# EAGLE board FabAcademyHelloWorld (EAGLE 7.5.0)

Size 100 x 80 mm. Coordinates in mm from the lower left corner, seen from the top.
Outline: 0,0 100,0 100,80 0,80 0,0
Copper layers (1*16): Top 0.035mm / dielectric 1.5mm / Bottom 0.035mm
Design rules "default": minimum track width 10mil, minimum drill 24mil, track to track 8mil, track to pad 8mil, pad to pad 8mil, via to via 8mil, smd to smd 8mil, copper to edge 40mil, drill to drill 8mil, minimum pad ring 10mil, minimum via ring 8mil, stop-mask expansion 4mil, vias tented up to drill 0mil, thermal gap 10mil

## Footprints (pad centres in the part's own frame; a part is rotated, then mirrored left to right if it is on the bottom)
C1206FAB = smd 1.27 x 1.905: 1 -1.651,0; 2 1.651,0
SOIC14 = smd 0.61 x 2.21: 1 -3.81,-2.603; 2 -2.54,-2.603; 3 -1.27,-2.603; 4 0,-2.603; 5 1.27,-2.603; 6 2.54,-2.603; 7 3.81,-2.603; 8 3.81,2.603; 9 2.54,2.603; 10 1.27,2.603; 11 0,2.603; 12 -1.27,2.603; 13 -2.54,2.603; 14 -3.81,2.603
1X02 = drill 1.016 pad 1.88: 1 0,0; 2 2.54,0
R1206FAB = smd 1.27 x 1.905: 1 -1.651,0; 2 1.651,0
6MM_SWITCH = smd 2.286 x 1.524: 1 -3.302,2.286; 2 3.302,2.286; 3 -3.302,-2.286; 4 3.302,-2.286
2X03SMD = smd 2.54 x 1.27: 1 -2.54,2.54; 2 2.92,2.54; 3 -2.54,0; 4 2.92,0; 5 -2.54,-2.54; 6 2.92,-2.54
1X06SMD = smd 2.54 x 1.27: 1 0,6.35; 2 0,3.81; 3 0,1.27; 4 0,-1.27; 5 0,-3.81; 6 0,-6.35
EFOBM = smd 0.8 x 3.9: 1 -1.35,0; 2 0,0; 3 1.35,0
LED1206FAB = smd 1.27 x 1.905: 1 -1.651,0; 2 1.651,0

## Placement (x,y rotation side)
C1  1uF  [C1206FAB]  25.4,54.61 0 top
IC1  ATTINY44-SSU  [SOIC14]  21.59,46.99 270 top
JP1  [1X02]  40.64,44.45 270 top
R1  499  [R1206FAB]  13.97,45.72 180 top
R2  10k  [R1206FAB]  30.48,41.91 180 top
R3  10k  [R1206FAB]  20.32,54.61 180 top
S1  [6MM_SWITCH]  31.75,35.56 0 top
U$1  AVRISPSMD  [2X03SMD]  21.59,36.83 270 top
U$2  FTDI-SMD-HEADER  [1X06SMD]  40.64,53.34 180 top
U$3  20MHz  [EFOBM]  13.97,50.8 270 top
U$4  LEDFAB1206  [LED1206FAB]  13.97,41.91 180 top

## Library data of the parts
C1 IC1 R1-R3 S1 U$1-U$4 = fablab
JP1 = SparkFun-Connectors

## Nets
BUTTON: IC1.6
CTS: U$2.2
GND: C1.2 IC1.14 R1.1 S1.3 U$1.6 U$2.1 U$3.2
LED: IC1.5 U$4.1
MISO: IC1.8 U$1.1
MOSI: IC1.7 U$1.4
N$1: R1.2 U$4.2
N$2: IC1.2 U$3.1
N$3: IC1.11 JP1.1
N$4: IC1.10 JP1.2
N$5: R3.1 S1.1
N$9: IC1.3 U$3.3
RESET: IC1.4 R2.1 U$1.5
RTS: U$2.6
RX: IC1.12 U$2.5
SCK: IC1.9 U$1.3
TX: IC1.13 U$2.4
VCC: C1.1 IC1.1 R2.2 R3.2 U$1.2 U$2.3

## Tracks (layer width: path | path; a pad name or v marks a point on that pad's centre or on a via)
GND  (6 unrouted)
LED  (1 unrouted)
MISO  (1 unrouted)
MOSI  (1 unrouted)
N$1  (1 unrouted)
N$2  (1 unrouted)
N$3  (1 unrouted)
N$4  (1 unrouted)
N$5  (1 unrouted)
N$9  (1 unrouted)
RESET  (2 unrouted)
RX  (1 unrouted)
SCK  (1 unrouted)
TX  (1 unrouted)
VCC  (5 unrouted)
